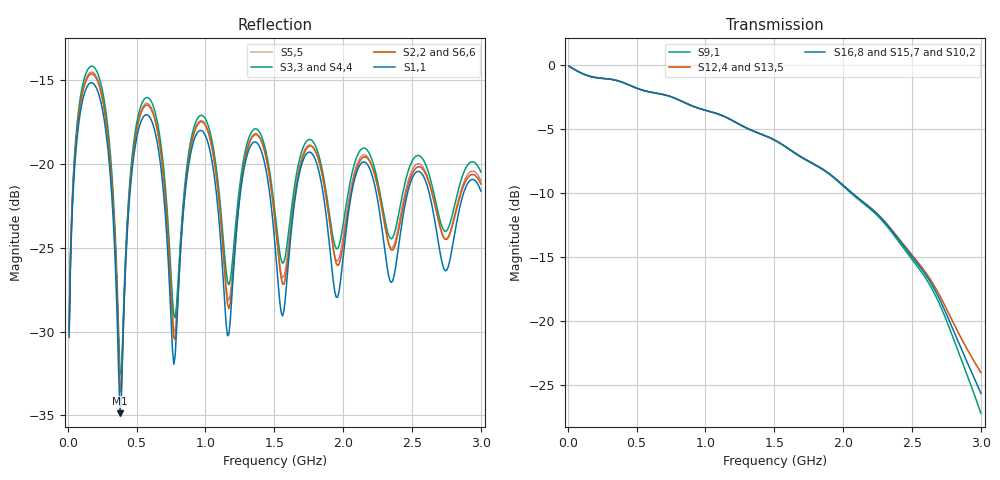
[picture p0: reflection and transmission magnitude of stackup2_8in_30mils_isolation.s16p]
! Touchstone file from project
# GHZ S RI R 50.000000
! Modal data exported
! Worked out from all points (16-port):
!   300 points, 10 MHz to 3 GHz, reference 50 ohm
!   strongest paths, dB at 10 MHz, 760 MHz, 1.51 GHz, 2.26 GHz, 3 GHz:
!     S16,8: -0.1, -2.5, -5.9, -11.8, -25.6
!     S12,4: -0.1, -2.5, -5.9, -11.7, -24.0
!     S15,7: -0.1, -2.5, -5.9, -11.8, -25.3
!     S13,5: -0.1, -2.5, -5.9, -11.8, -24.7
!     S9,1: -0.1, -2.5, -5.9, -11.9, -27.2
!     S10,2: -0.1, -2.5, -5.9, -11.9, -24.4
!   lowest |S11| = -34.9 dB at 380 MHz (marker M1), VSWR 1.04, Z = 51.8 - j0.555 ohm
!   |S11| at or under -10 dB: start of sweep to end of sweep
